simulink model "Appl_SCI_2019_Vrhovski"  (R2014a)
settings: Solver=ode45  StartTime=0.0  StopTime=1000  MaxStep=0.01  RelTol=1e-3
undefined symbols (not defined in the file): deg, H, kg, m, M, mm, N, rad, s, X, Y, Z
libraries: sm_lib x389, nesl_utility x69, simulink x7
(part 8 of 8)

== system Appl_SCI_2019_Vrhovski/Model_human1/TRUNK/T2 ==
  Mux : Mux  Inputs=3
  Pos X Converter : nesl_utility/PS-Simulink Converter  PhysicalDomain=network_engine_domain  SubClassName=ps_output  LeftPortType=input  RightPortType=output  PseudoPeriodic=off  Frequencies=[]  Unit=mm  AffineConversion=off
  Pos Y Converter : nesl_utility/PS-Simulink Converter  PhysicalDomain=network_engine_domain  SubClassName=ps_output  LeftPortType=input  RightPortType=output  PseudoPeriodic=off  Frequencies=[]  Unit=mm  AffineConversion=off
  Pos Z Converter2 : nesl_utility/PS-Simulink Converter  PhysicalDomain=network_engine_domain  SubClassName=ps_output  LeftPortType=input  RightPortType=output  PseudoPeriodic=off  Frequencies=[]  Unit=mm  AffineConversion=off
  Transform Sensor : sm_lib/Frames and Transforms/Transform Sensor  MeasurementFrame=World  SenseAngle=off  SenseAxis=off  SenseAngle1=off  SenseAngle2=off  SenseAngle3=off  SenseQ=off  SenseR=off  SenseOmegaX=off  SenseOmegaY=off  SenseOmegaZ=off  SenseOmega1=off  SenseOmega2=off  SenseOmega3=off  SenseQDot=off  SenseRDot=off  SenseAlphaX=off  SenseAlphaY=off  SenseAlphaZ=off  SenseAlpha1=off  SenseAlpha2=off  SenseAlpha3=off  SenseQDDot=off  SenseRDDot=off  SenseX=on  SenseY=on  SenseZ=on  SenseRad=on  SenseAzim=off  SenseDist=off  SenseInc=off  SenseXDot=off  SenseYDot=off  SenseZDot=off  SenseRadDot=off  SenseAzimDot=off  SenseDistDot=off  SenseIncDot=off  SenseXDDot=off  SenseYDDot=off  SenseZDDot=off  SenseRadDDot=off  SenseAzimDDot=off  SenseDistDDot=off  SenseIncDDot=off  BlockFunction=simmechanics.library.frames_transforms.transform_sensor
  base_coord_sys : PMIOPort  Port=1  Side=Left
  marker : PMIOPort  Port=2  Side=Left
  xyz : Outport
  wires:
  Mux/1 -> xyz/1
  Pos Y Converter/1 -> Mux/2
  Pos X Converter/1 -> Mux/1
  Pos Z Converter2/1 -> Mux/3
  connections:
  Transform Sensor/RConn3 -- Pos Y Converter/LConn1
  Pos X Converter/LConn1 -- Transform Sensor/RConn2
  Pos Z Converter2/LConn1 -- Transform Sensor/RConn4
  marker/RConn1 -- Transform Sensor/RConn1
  base_coord_sys/RConn1 -- Transform Sensor/LConn1

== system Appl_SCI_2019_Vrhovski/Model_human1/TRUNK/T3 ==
  Mux : Mux  Inputs=3
  Pos X Converter : nesl_utility/PS-Simulink Converter  PhysicalDomain=network_engine_domain  SubClassName=ps_output  LeftPortType=input  RightPortType=output  PseudoPeriodic=off  Frequencies=[]  Unit=mm  AffineConversion=off
  Pos Y Converter : nesl_utility/PS-Simulink Converter  PhysicalDomain=network_engine_domain  SubClassName=ps_output  LeftPortType=input  RightPortType=output  PseudoPeriodic=off  Frequencies=[]  Unit=mm  AffineConversion=off
  Pos Z Converter2 : nesl_utility/PS-Simulink Converter  PhysicalDomain=network_engine_domain  SubClassName=ps_output  LeftPortType=input  RightPortType=output  PseudoPeriodic=off  Frequencies=[]  Unit=mm  AffineConversion=off
  Transform Sensor : sm_lib/Frames and Transforms/Transform Sensor  MeasurementFrame=World  SenseAngle=off  SenseAxis=off  SenseAngle1=off  SenseAngle2=off  SenseAngle3=off  SenseQ=off  SenseR=off  SenseOmegaX=off  SenseOmegaY=off  SenseOmegaZ=off  SenseOmega1=off  SenseOmega2=off  SenseOmega3=off  SenseQDot=off  SenseRDot=off  SenseAlphaX=off  SenseAlphaY=off  SenseAlphaZ=off  SenseAlpha1=off  SenseAlpha2=off  SenseAlpha3=off  SenseQDDot=off  SenseRDDot=off  SenseX=on  SenseY=on  SenseZ=on  SenseRad=on  SenseAzim=off  SenseDist=off  SenseInc=off  SenseXDot=off  SenseYDot=off  SenseZDot=off  SenseRadDot=off  SenseAzimDot=off  SenseDistDot=off  SenseIncDot=off  SenseXDDot=off  SenseYDDot=off  SenseZDDot=off  SenseRadDDot=off  SenseAzimDDot=off  SenseDistDDot=off  SenseIncDDot=off  BlockFunction=simmechanics.library.frames_transforms.transform_sensor
  base_coord_sys : PMIOPort  Port=1  Side=Left
  marker : PMIOPort  Port=2  Side=Left
  xyz : Outport
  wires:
  Pos Z Converter2/1 -> Mux/3
  Pos X Converter/1 -> Mux/1
  Pos Y Converter/1 -> Mux/2
  Mux/1 -> xyz/1
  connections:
  base_coord_sys/RConn1 -- Transform Sensor/LConn1
  marker/RConn1 -- Transform Sensor/RConn1
  Pos Z Converter2/LConn1 -- Transform Sensor/RConn4
  Pos X Converter/LConn1 -- Transform Sensor/RConn2
  Transform Sensor/RConn3 -- Pos Y Converter/LConn1

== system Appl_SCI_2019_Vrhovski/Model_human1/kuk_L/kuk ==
  ReferenceFrame : sm_lib/Frames and Transforms/Reference Frame  BlockFunction=simmechanics.library.frames_transforms.reference_frame
  Solid : sm_lib/Body Elements/Solid  InertiaType=Custom  Mass=0  MassUnits=kg  CenterOfMass=[0 0 0]  CenterOfMassUnits=mm  MomentsOfInertia=[2897.1863857204326 1.8962829928219973 2897.1862300567827]  MomentsOfInertiaUnits=kg*mm^2  ProductsOfInertia=[0 0 -0.00027890183916846033]  ProductsOfInertiaUnits=kg*mm^2  DensityBased=on  Density=1000  DensityUnits=kg/(m^3)  GraphicType=FromGeometry  MarkerShape=Sphere  MarkerSize=10  MarkerSizeUnits=m  GraphicVisPropType=SimpleVisualProperties  GraphicDiffuseColor=[0.792156862745098 0.81960784313725488 0.93333333333333335]  GraphicSpecularColor=[0.5 0.5 0.5 1.0]  GraphicAmbientColor=[0.15 0.15 0.15 1.0]  GraphicEmissiveColor=[0.0 0.0 0.0 1.0]  GraphicShininess=75  GraphicOpacity=1  GeometryShape=Sphere  RectangleSize=[1 1]  RectangleSizeUnits=m  BrickDimensions=[1 1 1]  BrickDimensionUnits=m  CylinderRadius=1  CylinderRadiusUnits=m  CylinderLength=1  CylinderLengthUnits=m  SphereRadius=3  SphereRadiusUnits=cm  EllipsoidRadii=[1 1 1]  EllipsoidRadiiUnits=m  ExtrusionCrossSection=[1 1; -1 1; -1 -1; 1 -1]  ExtrusionCrossSectionUnits=m  ExtrusionLength=1  ExtrusionLengthUnits=m  PolygonNumSides=3  PolygonOuterRadius=1  PolygonOuterRadiusUnits=m  ExtGeomFileType=STL  ExtGeomFileName=Pod_Default_sldprt.STL  ExtGeomFileUnits=mm  RevolutionCrossSection=[1 1; 1 -1; 2 -1; 2 1]  RevolutionCrossSectionUnits=m  RevolutionExtent=Full  RevolutionAngle=180  RevolutionAngleUnits=deg  BlockFunction=simmechanics.library.body_elements.solid
  Transform : sm_lib/Frames and Transforms/Rigid Transform  TranslationMethod=None  TranslationLengthUnit=mm  TranslationStandardAxis=+Z  TranslationStandardOffset=100  TranslationCartesianOffset=[-2.2026824808563106e-13 549.99999999999943 3.4106051316484809e-13]  TranslationROffset=0  TranslationROffsetUnits=m  TranslationZOffset=0  TranslationZOffsetUnits=m  TranslationThetaOffset=0  TranslationThetaOffsetUnits=deg  RotationMethod=None  RotationAngleUnits=rad  RotationStandardAxis=+Z  RotationAngle=2.0943951023931962  RotationArbitraryAxis=[0.57735026918962595 -0.57735026918962618 0.57735026918962518]  FollAlignAxisA=+X  BaseAlignAxisA=+Y  FollAlignAxisB=+Y  BaseAlignAxisB=+Z  BlockFunction=simmechanics.library.frames_transforms.rigid_transform
  Transform1 : sm_lib/Frames and Transforms/Rigid Transform  TranslationMethod=StandardAxis  TranslationLengthUnit=mm  TranslationStandardAxis=+Z  TranslationStandardOffset=50  TranslationCartesianOffset=[1.3358203432289883e-12 0 -1.0913936421275139e-11]  TranslationROffset=0  TranslationROffsetUnits=m  TranslationZOffset=0  TranslationZOffsetUnits=m  TranslationThetaOffset=0  TranslationThetaOffsetUnits=deg  RotationMethod=None  RotationAngleUnits=rad  RotationStandardAxis=+X  RotationAngle=pi/2  RotationArbitraryAxis=[0 0 0]  FollAlignAxisA=+X  BaseAlignAxisA=+Y  FollAlignAxisB=+Y  BaseAlignAxisB=+Z  BlockFunction=simmechanics.library.frames_transforms.rigid_transform
  F : PMIOPort  Port=1  Side=Right
  B : PMIOPort  Port=2  Side=Left
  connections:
  Transform1/RConn1 -- F/RConn1
  Transform/RConn1 -- B/RConn1
  Solid/RConn1 -- ReferenceFrame/RConn1 -- Transform1/LConn1 -- Transform/LConn1

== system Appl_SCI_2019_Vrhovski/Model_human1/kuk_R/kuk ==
  ReferenceFrame : sm_lib/Frames and Transforms/Reference Frame  BlockFunction=simmechanics.library.frames_transforms.reference_frame
  Solid : sm_lib/Body Elements/Solid  InertiaType=Custom  Mass=0  MassUnits=kg  CenterOfMass=[0 0 0]  CenterOfMassUnits=mm  MomentsOfInertia=[2897.1863857204326 1.8962829928219973 2897.1862300567827]  MomentsOfInertiaUnits=kg*mm^2  ProductsOfInertia=[0 0 -0.00027890183916846033]  ProductsOfInertiaUnits=kg*mm^2  DensityBased=on  Density=1000  DensityUnits=kg/(m^3)  GraphicType=FromGeometry  MarkerShape=Sphere  MarkerSize=10  MarkerSizeUnits=m  GraphicVisPropType=SimpleVisualProperties  GraphicDiffuseColor=[0.792156862745098 0.81960784313725488 0.93333333333333335]  GraphicSpecularColor=[0.5 0.5 0.5 1.0]  GraphicAmbientColor=[0.15 0.15 0.15 1.0]  GraphicEmissiveColor=[0.0 0.0 0.0 1.0]  GraphicShininess=75  GraphicOpacity=1  GeometryShape=Sphere  RectangleSize=[1 1]  RectangleSizeUnits=m  BrickDimensions=[1 1 1]  BrickDimensionUnits=m  CylinderRadius=1  CylinderRadiusUnits=m  CylinderLength=1  CylinderLengthUnits=m  SphereRadius=3  SphereRadiusUnits=cm  EllipsoidRadii=[1 1 1]  EllipsoidRadiiUnits=m  ExtrusionCrossSection=[1 1; -1 1; -1 -1; 1 -1]  ExtrusionCrossSectionUnits=m  ExtrusionLength=1  ExtrusionLengthUnits=m  PolygonNumSides=3  PolygonOuterRadius=1  PolygonOuterRadiusUnits=m  ExtGeomFileType=STL  ExtGeomFileName=Pod_Default_sldprt.STL  ExtGeomFileUnits=mm  RevolutionCrossSection=[1 1; 1 -1; 2 -1; 2 1]  RevolutionCrossSectionUnits=m  RevolutionExtent=Full  RevolutionAngle=180  RevolutionAngleUnits=deg  BlockFunction=simmechanics.library.body_elements.solid
  Transform : sm_lib/Frames and Transforms/Rigid Transform  TranslationMethod=None  TranslationLengthUnit=mm  TranslationStandardAxis=+Z  TranslationStandardOffset=0  TranslationCartesianOffset=[-2.2026824808563106e-13 549.99999999999943 3.4106051316484809e-13]  TranslationROffset=0  TranslationROffsetUnits=m  TranslationZOffset=0  TranslationZOffsetUnits=m  TranslationThetaOffset=0  TranslationThetaOffsetUnits=deg  RotationMethod=None  RotationAngleUnits=rad  RotationStandardAxis=+Z  RotationAngle=2.0943951023931962  RotationArbitraryAxis=[0.57735026918962595 -0.57735026918962618 0.57735026918962518]  FollAlignAxisA=+X  BaseAlignAxisA=+Y  FollAlignAxisB=+Y  BaseAlignAxisB=+Z  BlockFunction=simmechanics.library.frames_transforms.rigid_transform
  Transform1 : sm_lib/Frames and Transforms/Rigid Transform  TranslationMethod=StandardAxis  TranslationLengthUnit=mm  TranslationStandardAxis=+Z  TranslationStandardOffset=50  TranslationCartesianOffset=[1.3358203432289883e-12 0 -1.0913936421275139e-11]  TranslationROffset=0  TranslationROffsetUnits=m  TranslationZOffset=0  TranslationZOffsetUnits=m  TranslationThetaOffset=0  TranslationThetaOffsetUnits=deg  RotationMethod=None  RotationAngleUnits=rad  RotationStandardAxis=+X  RotationAngle=pi/2  RotationArbitraryAxis=[0 0 0]  FollAlignAxisA=+X  BaseAlignAxisA=+Y  FollAlignAxisB=+Y  BaseAlignAxisB=+Z  BlockFunction=simmechanics.library.frames_transforms.rigid_transform
  F : PMIOPort  Port=1  Side=Right
  B : PMIOPort  Port=2  Side=Left
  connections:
  Transform/LConn1 -- Transform1/LConn1 -- ReferenceFrame/RConn1 -- Solid/RConn1
  Transform/RConn1 -- B/RConn1
  Transform1/RConn1 -- F/RConn1

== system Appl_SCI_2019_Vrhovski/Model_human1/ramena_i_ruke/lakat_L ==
  ReferenceFrame : sm_lib/Frames and Transforms/Reference Frame  BlockFunction=simmechanics.library.frames_transforms.reference_frame
  Solid : sm_lib/Body Elements/Solid  InertiaType=Custom  Mass=0  MassUnits=kg  CenterOfMass=[0 0 0]  CenterOfMassUnits=mm  MomentsOfInertia=[2897.1863857204326 1.8962829928219973 2897.1862300567827]  MomentsOfInertiaUnits=kg*mm^2  ProductsOfInertia=[0 0 -0.00027890183916846033]  ProductsOfInertiaUnits=kg*mm^2  DensityBased=on  Density=1000  DensityUnits=kg/(m^3)  GraphicType=FromGeometry  MarkerShape=Sphere  MarkerSize=10  MarkerSizeUnits=m  GraphicVisPropType=SimpleVisualProperties  GraphicDiffuseColor=[0.792156862745098 0.81960784313725488 0.93333333333333335]  GraphicSpecularColor=[0.5 0.5 0.5 1.0]  GraphicAmbientColor=[0.15 0.15 0.15 1.0]  GraphicEmissiveColor=[0.0 0.0 0.0 1.0]  GraphicShininess=75  GraphicOpacity=1  GeometryShape=Sphere  RectangleSize=[1 1]  RectangleSizeUnits=m  BrickDimensions=[1 1 1]  BrickDimensionUnits=m  CylinderRadius=1  CylinderRadiusUnits=m  CylinderLength=1  CylinderLengthUnits=m  SphereRadius=3  SphereRadiusUnits=cm  EllipsoidRadii=[1 1 1]  EllipsoidRadiiUnits=m  ExtrusionCrossSection=[1 1; -1 1; -1 -1; 1 -1]  ExtrusionCrossSectionUnits=m  ExtrusionLength=1  ExtrusionLengthUnits=m  PolygonNumSides=3  PolygonOuterRadius=1  PolygonOuterRadiusUnits=m  ExtGeomFileType=STL  ExtGeomFileName=Pod_Default_sldprt.STL  ExtGeomFileUnits=mm  RevolutionCrossSection=[1 1; 1 -1; 2 -1; 2 1]  RevolutionCrossSectionUnits=m  RevolutionExtent=Full  RevolutionAngle=180  RevolutionAngleUnits=deg  BlockFunction=simmechanics.library.body_elements.solid
  Transform : sm_lib/Frames and Transforms/Rigid Transform  TranslationMethod=None  TranslationLengthUnit=mm  TranslationStandardAxis=+Z  TranslationStandardOffset=0  TranslationCartesianOffset=[-2.2026824808563106e-13 549.99999999999943 3.4106051316484809e-13]  TranslationROffset=0  TranslationROffsetUnits=m  TranslationZOffset=0  TranslationZOffsetUnits=m  TranslationThetaOffset=0  TranslationThetaOffsetUnits=deg  RotationMethod=None  RotationAngleUnits=rad  RotationStandardAxis=+Z  RotationAngle=2.0943951023931962  RotationArbitraryAxis=[0.57735026918962595 -0.57735026918962618 0.57735026918962518]  FollAlignAxisA=+X  BaseAlignAxisA=+Y  FollAlignAxisB=+Y  BaseAlignAxisB=+Z  BlockFunction=simmechanics.library.frames_transforms.rigid_transform
  Transform1 : sm_lib/Frames and Transforms/Rigid Transform  TranslationMethod=None  TranslationLengthUnit=mm  TranslationStandardAxis=+Z  TranslationStandardOffset=0  TranslationCartesianOffset=[1.3358203432289883e-12 0 -1.0913936421275139e-11]  TranslationROffset=0  TranslationROffsetUnits=m  TranslationZOffset=0  TranslationZOffsetUnits=m  TranslationThetaOffset=0  TranslationThetaOffsetUnits=deg  RotationMethod=None  RotationAngleUnits=rad  RotationStandardAxis=+X  RotationAngle=pi/2  RotationArbitraryAxis=[0 0 0]  FollAlignAxisA=+X  BaseAlignAxisA=+Y  FollAlignAxisB=+Y  BaseAlignAxisB=+Z  BlockFunction=simmechanics.library.frames_transforms.rigid_transform
  F : PMIOPort  Port=1  Side=Right
  B : PMIOPort  Port=2  Side=Left
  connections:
  Transform/LConn1 -- Transform1/LConn1 -- ReferenceFrame/RConn1 -- Solid/RConn1
  Transform/RConn1 -- B/RConn1
  Transform1/RConn1 -- F/RConn1

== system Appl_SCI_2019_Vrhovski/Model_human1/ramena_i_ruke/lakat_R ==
  ReferenceFrame : sm_lib/Frames and Transforms/Reference Frame  BlockFunction=simmechanics.library.frames_transforms.reference_frame
  Solid : sm_lib/Body Elements/Solid  InertiaType=Custom  Mass=0  MassUnits=kg  CenterOfMass=[0 0 0]  CenterOfMassUnits=mm  MomentsOfInertia=[2897.1863857204326 1.8962829928219973 2897.1862300567827]  MomentsOfInertiaUnits=kg*mm^2  ProductsOfInertia=[0 0 -0.00027890183916846033]  ProductsOfInertiaUnits=kg*mm^2  DensityBased=on  Density=1000  DensityUnits=kg/(m^3)  GraphicType=FromGeometry  MarkerShape=Sphere  MarkerSize=10  MarkerSizeUnits=m  GraphicVisPropType=SimpleVisualProperties  GraphicDiffuseColor=[0.792156862745098 0.81960784313725488 0.93333333333333335]  GraphicSpecularColor=[0.5 0.5 0.5 1.0]  GraphicAmbientColor=[0.15 0.15 0.15 1.0]  GraphicEmissiveColor=[0.0 0.0 0.0 1.0]  GraphicShininess=75  GraphicOpacity=1  GeometryShape=Sphere  RectangleSize=[1 1]  RectangleSizeUnits=m  BrickDimensions=[1 1 1]  BrickDimensionUnits=m  CylinderRadius=1  CylinderRadiusUnits=m  CylinderLength=1  CylinderLengthUnits=m  SphereRadius=3  SphereRadiusUnits=cm  EllipsoidRadii=[1 1 1]  EllipsoidRadiiUnits=m  ExtrusionCrossSection=[1 1; -1 1; -1 -1; 1 -1]  ExtrusionCrossSectionUnits=m  ExtrusionLength=1  ExtrusionLengthUnits=m  PolygonNumSides=3  PolygonOuterRadius=1  PolygonOuterRadiusUnits=m  ExtGeomFileType=STL  ExtGeomFileName=Pod_Default_sldprt.STL  ExtGeomFileUnits=mm  RevolutionCrossSection=[1 1; 1 -1; 2 -1; 2 1]  RevolutionCrossSectionUnits=m  RevolutionExtent=Full  RevolutionAngle=180  RevolutionAngleUnits=deg  BlockFunction=simmechanics.library.body_elements.solid
  Transform : sm_lib/Frames and Transforms/Rigid Transform  TranslationMethod=None  TranslationLengthUnit=mm  TranslationStandardAxis=+Z  TranslationStandardOffset=0  TranslationCartesianOffset=[-2.2026824808563106e-13 549.99999999999943 3.4106051316484809e-13]  TranslationROffset=0  TranslationROffsetUnits=m  TranslationZOffset=0  TranslationZOffsetUnits=m  TranslationThetaOffset=0  TranslationThetaOffsetUnits=deg  RotationMethod=None  RotationAngleUnits=rad  RotationStandardAxis=+Z  RotationAngle=2.0943951023931962  RotationArbitraryAxis=[0.57735026918962595 -0.57735026918962618 0.57735026918962518]  FollAlignAxisA=+X  BaseAlignAxisA=+Y  FollAlignAxisB=+Y  BaseAlignAxisB=+Z  BlockFunction=simmechanics.library.frames_transforms.rigid_transform
  Transform1 : sm_lib/Frames and Transforms/Rigid Transform  TranslationMethod=None  TranslationLengthUnit=mm  TranslationStandardAxis=+Z  TranslationStandardOffset=0  TranslationCartesianOffset=[1.3358203432289883e-12 0 -1.0913936421275139e-11]  TranslationROffset=0  TranslationROffsetUnits=m  TranslationZOffset=0  TranslationZOffsetUnits=m  TranslationThetaOffset=0  TranslationThetaOffsetUnits=deg  RotationMethod=None  RotationAngleUnits=rad  RotationStandardAxis=+X  RotationAngle=pi/2  RotationArbitraryAxis=[0 0 0]  FollAlignAxisA=+X  BaseAlignAxisA=+Y  FollAlignAxisB=+Y  BaseAlignAxisB=+Z  BlockFunction=simmechanics.library.frames_transforms.rigid_transform
  F : PMIOPort  Port=1  Side=Right
  B : PMIOPort  Port=2  Side=Left
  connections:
  Transform1/RConn1 -- F/RConn1
  Transform/RConn1 -- B/RConn1
  Solid/RConn1 -- ReferenceFrame/RConn1 -- Transform1/LConn1 -- Transform/LConn1

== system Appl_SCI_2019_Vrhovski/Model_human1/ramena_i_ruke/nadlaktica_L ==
  ReferenceFrame : sm_lib/Frames and Transforms/Reference Frame  BlockFunction=simmechanics.library.frames_transforms.reference_frame
  Solid : sm_lib/Body Elements/Solid  InertiaType=Custom  Mass=0.03*M  MassUnits=kg  CenterOfMass=[0 0 0]  CenterOfMassUnits=mm  MomentsOfInertia=[2897.1863857204326 1.8962829928219973 2897.1862300567827]  MomentsOfInertiaUnits=kg*mm^2  ProductsOfInertia=[0 0 -0.00027890183916846033]  ProductsOfInertiaUnits=kg*mm^2  DensityBased=on  Density=1000  DensityUnits=kg/(m^3)  GraphicType=FromGeometry  MarkerShape=Sphere  MarkerSize=10  MarkerSizeUnits=m  GraphicVisPropType=SimpleVisualProperties  GraphicDiffuseColor=[0.792156862745098 0.81960784313725488 0.93333333333333335]  GraphicSpecularColor=[0.5 0.5 0.5 1.0]  GraphicAmbientColor=[0.15 0.15 0.15 1.0]  GraphicEmissiveColor=[0.0 0.0 0.0 1.0]  GraphicShininess=75  GraphicOpacity=1  GeometryShape=Ellipsoid  RectangleSize=[1 1]  RectangleSizeUnits=m  BrickDimensions=[1 1 1]  BrickDimensionUnits=m  CylinderRadius=2.5  CylinderRadiusUnits=cm  CylinderLength=25  CylinderLengthUnits=cm  SphereRadius=5  SphereRadiusUnits=cm  EllipsoidRadii=[40 40 125]  EllipsoidRadiiUnits=mm  ExtrusionCrossSection=[1 1; -1 1; -1 -1; 1 -1]  ExtrusionCrossSectionUnits=m  ExtrusionLength=1  ExtrusionLengthUnits=m  PolygonNumSides=3  PolygonOuterRadius=1  PolygonOuterRadiusUnits=m  ExtGeomFileType=STL  ExtGeomFileName=Pod_Default_sldprt.STL  ExtGeomFileUnits=mm  RevolutionCrossSection=[1 1; 1 -1; 2 -1; 2 1]  RevolutionCrossSectionUnits=m  RevolutionExtent=Full  RevolutionAngle=180  RevolutionAngleUnits=deg  BlockFunction=simmechanics.library.body_elements.solid
  Transform1 : sm_lib/Frames and Transforms/Rigid Transform  TranslationMethod=StandardAxis  TranslationLengthUnit=mm  TranslationStandardAxis=+Z  TranslationStandardOffset=125  TranslationCartesianOffset=[1.3358203432289883e-12 650.00000000000045 -1.0913936421275139e-11]  TranslationROffset=0  TranslationROffsetUnits=m  TranslationZOffset=0  TranslationZOffsetUnits=m  TranslationThetaOffset=0  TranslationThetaOffsetUnits=deg  RotationMethod=None  RotationAngleUnits=rad  RotationStandardAxis=+Z  RotationAngle=0  RotationArbitraryAxis=[0 0 0]  FollAlignAxisA=+X  BaseAlignAxisA=+Y  FollAlignAxisB=+Y  BaseAlignAxisB=+Z  BlockFunction=simmechanics.library.frames_transforms.rigid_transform
  Transform2 : sm_lib/Frames and Transforms/Rigid Transform  TranslationMethod=StandardAxis  TranslationLengthUnit=mm  TranslationStandardAxis=-Z  TranslationStandardOffset=125  TranslationCartesianOffset=[-2.2026824808563106e-13 549.99999999999943 3.4106051316484809e-13]  TranslationROffset=0  TranslationROffsetUnits=m  TranslationZOffset=0  TranslationZOffsetUnits=m  TranslationThetaOffset=0  TranslationThetaOffsetUnits=deg  RotationMethod=None  RotationAngleUnits=rad  RotationStandardAxis=+X  RotationAngle=pi/2  RotationArbitraryAxis=[0.57735026918962595 -0.57735026918962618 0.57735026918962518]  FollAlignAxisA=+X  BaseAlignAxisA=+Y  FollAlignAxisB=+Y  BaseAlignAxisB=+Z  BlockFunction=simmechanics.library.frames_transforms.rigid_transform
  F : PMIOPort  Port=1  Side=Right
  B : PMIOPort  Port=2  Side=Left
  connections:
  Transform2/LConn1 -- Transform1/LConn1 -- Solid/RConn1 -- ReferenceFrame/RConn1
  Transform1/RConn1 -- F/RConn1
  B/RConn1 -- Transform2/RConn1

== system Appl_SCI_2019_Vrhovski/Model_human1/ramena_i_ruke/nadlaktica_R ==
  ReferenceFrame : sm_lib/Frames and Transforms/Reference Frame  BlockFunction=simmechanics.library.frames_transforms.reference_frame
  Solid : sm_lib/Body Elements/Solid  InertiaType=Custom  Mass=0.03*M  MassUnits=kg  CenterOfMass=[0 0 0]  CenterOfMassUnits=mm  MomentsOfInertia=[2897.1863857204326 1.8962829928219973 2897.1862300567827]  MomentsOfInertiaUnits=kg*mm^2  ProductsOfInertia=[0 0 -0.00027890183916846033]  ProductsOfInertiaUnits=kg*mm^2  DensityBased=on  Density=1000  DensityUnits=kg/(m^3)  GraphicType=FromGeometry  MarkerShape=Sphere  MarkerSize=10  MarkerSizeUnits=m  GraphicVisPropType=SimpleVisualProperties  GraphicDiffuseColor=[0.792156862745098 0.81960784313725488 0.93333333333333335]  GraphicSpecularColor=[0.5 0.5 0.5 1.0]  GraphicAmbientColor=[0.15 0.15 0.15 1.0]  GraphicEmissiveColor=[0.0 0.0 0.0 1.0]  GraphicShininess=75  GraphicOpacity=1  GeometryShape=Ellipsoid  RectangleSize=[1 1]  RectangleSizeUnits=m  BrickDimensions=[1 1 1]  BrickDimensionUnits=m  CylinderRadius=2.5  CylinderRadiusUnits=cm  CylinderLength=25  CylinderLengthUnits=cm  SphereRadius=5  SphereRadiusUnits=cm  EllipsoidRadii=[40 40 125]  EllipsoidRadiiUnits=mm  ExtrusionCrossSection=[1 1; -1 1; -1 -1; 1 -1]  ExtrusionCrossSectionUnits=m  ExtrusionLength=1  ExtrusionLengthUnits=m  PolygonNumSides=3  PolygonOuterRadius=1  PolygonOuterRadiusUnits=m  ExtGeomFileType=STL  ExtGeomFileName=Pod_Default_sldprt.STL  ExtGeomFileUnits=mm  RevolutionCrossSection=[1 1; 1 -1; 2 -1; 2 1]  RevolutionCrossSectionUnits=m  RevolutionExtent=Full  RevolutionAngle=180  RevolutionAngleUnits=deg  BlockFunction=simmechanics.library.body_elements.solid
  Transform1 : sm_lib/Frames and Transforms/Rigid Transform  TranslationMethod=StandardAxis  TranslationLengthUnit=mm  TranslationStandardAxis=+Z  TranslationStandardOffset=125  TranslationCartesianOffset=[1.3358203432289883e-12 650.00000000000045 -1.0913936421275139e-11]  TranslationROffset=0  TranslationROffsetUnits=m  TranslationZOffset=0  TranslationZOffsetUnits=m  TranslationThetaOffset=0  TranslationThetaOffsetUnits=deg  RotationMethod=None  RotationAngleUnits=rad  RotationStandardAxis=+Z  RotationAngle=0  RotationArbitraryAxis=[0 0 0]  FollAlignAxisA=+X  BaseAlignAxisA=+Y  FollAlignAxisB=+Y  BaseAlignAxisB=+Z  BlockFunction=simmechanics.library.frames_transforms.rigid_transform
  Transform2 : sm_lib/Frames and Transforms/Rigid Transform  TranslationMethod=StandardAxis  TranslationLengthUnit=mm  TranslationStandardAxis=-Z  TranslationStandardOffset=125  TranslationCartesianOffset=[-2.2026824808563106e-13 549.99999999999943 3.4106051316484809e-13]  TranslationROffset=0  TranslationROffsetUnits=m  TranslationZOffset=0  TranslationZOffsetUnits=m  TranslationThetaOffset=0  TranslationThetaOffsetUnits=deg  RotationMethod=None  RotationAngleUnits=rad  RotationStandardAxis=+X  RotationAngle=pi/2  RotationArbitraryAxis=[0.57735026918962595 -0.57735026918962618 0.57735026918962518]  FollAlignAxisA=+X  BaseAlignAxisA=+Y  FollAlignAxisB=+Y  BaseAlignAxisB=+Z  BlockFunction=simmechanics.library.frames_transforms.rigid_transform
  F : PMIOPort  Port=1  Side=Right
  B : PMIOPort  Port=2  Side=Left
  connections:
  B/RConn1 -- Transform2/RConn1
  Transform1/RConn1 -- F/RConn1
  ReferenceFrame/RConn1 -- Solid/RConn1 -- Transform1/LConn1 -- Transform2/LConn1

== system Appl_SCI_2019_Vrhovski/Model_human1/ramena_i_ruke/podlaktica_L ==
  ReferenceFrame : sm_lib/Frames and Transforms/Reference Frame  BlockFunction=simmechanics.library.frames_transforms.reference_frame
  Solid : sm_lib/Body Elements/Solid  InertiaType=Custom  Mass=0.0194*M  MassUnits=kg  CenterOfMass=[0 0 0]  CenterOfMassUnits=mm  MomentsOfInertia=[2897.1863857204326 1.8962829928219973 2897.1862300567827]  MomentsOfInertiaUnits=kg*mm^2  ProductsOfInertia=[0 0 -0.00027890183916846033]  ProductsOfInertiaUnits=kg*mm^2  DensityBased=on  Density=1000  DensityUnits=kg/(m^3)  GraphicType=FromGeometry  MarkerShape=Sphere  MarkerSize=10  MarkerSizeUnits=m  GraphicVisPropType=SimpleVisualProperties  GraphicDiffuseColor=[0.792156862745098 0.81960784313725488 0.93333333333333335]  GraphicSpecularColor=[0.5 0.5 0.5 1.0]  GraphicAmbientColor=[0.15 0.15 0.15 1.0]  GraphicEmissiveColor=[0.0 0.0 0.0 1.0]  GraphicShininess=75  GraphicOpacity=1  GeometryShape=Ellipsoid  RectangleSize=[1 1]  RectangleSizeUnits=m  BrickDimensions=[1 1 1]  BrickDimensionUnits=m  CylinderRadius=2.5  CylinderRadiusUnits=cm  CylinderLength=20  CylinderLengthUnits=cm  SphereRadius=5  SphereRadiusUnits=cm  EllipsoidRadii=[30 30 100]  EllipsoidRadiiUnits=mm  ExtrusionCrossSection=[1 1; -1 1; -1 -1; 1 -1]  ExtrusionCrossSectionUnits=m  ExtrusionLength=1  ExtrusionLengthUnits=m  PolygonNumSides=3  PolygonOuterRadius=1  PolygonOuterRadiusUnits=m  ExtGeomFileType=STL  ExtGeomFileName=Pod_Default_sldprt.STL  ExtGeomFileUnits=mm  RevolutionCrossSection=[1 1; 1 -1; 2 -1; 2 1]  RevolutionCrossSectionUnits=m  RevolutionExtent=Full  RevolutionAngle=180  RevolutionAngleUnits=deg  BlockFunction=simmechanics.library.body_elements.solid
  Transform1 : sm_lib/Frames and Transforms/Rigid Transform  TranslationMethod=StandardAxis  TranslationLengthUnit=mm  TranslationStandardAxis=+Z  TranslationStandardOffset=100  TranslationCartesianOffset=[1.3358203432289883e-12 650.00000000000045 -1.0913936421275139e-11]  TranslationROffset=0  TranslationROffsetUnits=m  TranslationZOffset=0  TranslationZOffsetUnits=m  TranslationThetaOffset=0  TranslationThetaOffsetUnits=deg  RotationMethod=None  RotationAngleUnits=rad  RotationStandardAxis=+Z  RotationAngle=0  RotationArbitraryAxis=[0 0 0]  FollAlignAxisA=+X  BaseAlignAxisA=+Y  FollAlignAxisB=+Y  BaseAlignAxisB=+Z  BlockFunction=simmechanics.library.frames_transforms.rigid_transform
  Transform2 : sm_lib/Frames and Transforms/Rigid Transform  TranslationMethod=StandardAxis  TranslationLengthUnit=mm  TranslationStandardAxis=-Z  TranslationStandardOffset=100  TranslationCartesianOffset=[-2.2026824808563106e-13 549.99999999999943 3.4106051316484809e-13]  TranslationROffset=0  TranslationROffsetUnits=m  TranslationZOffset=0  TranslationZOffsetUnits=m  TranslationThetaOffset=0  TranslationThetaOffsetUnits=deg  RotationMethod=None  RotationAngleUnits=rad  RotationStandardAxis=+X  RotationAngle=pi/2  RotationArbitraryAxis=[0.57735026918962595 -0.57735026918962618 0.57735026918962518]  FollAlignAxisA=+X  BaseAlignAxisA=+Y  FollAlignAxisB=+Y  BaseAlignAxisB=+Z  BlockFunction=simmechanics.library.frames_transforms.rigid_transform
  F : PMIOPort  Port=1  Side=Right
  B : PMIOPort  Port=2  Side=Left
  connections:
  B/RConn1 -- Transform2/RConn1
  Transform1/RConn1 -- F/RConn1
  ReferenceFrame/RConn1 -- Solid/RConn1 -- Transform1/LConn1 -- Transform2/LConn1

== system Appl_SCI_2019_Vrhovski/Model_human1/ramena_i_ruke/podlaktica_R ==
  ReferenceFrame : sm_lib/Frames and Transforms/Reference Frame  BlockFunction=simmechanics.library.frames_transforms.reference_frame
  Solid : sm_lib/Body Elements/Solid  InertiaType=Custom  Mass=0.0194*M  MassUnits=kg  CenterOfMass=[0 0 0]  CenterOfMassUnits=mm  MomentsOfInertia=[2897.1863857204326 1.8962829928219973 2897.1862300567827]  MomentsOfInertiaUnits=kg*mm^2  ProductsOfInertia=[0 0 -0.00027890183916846033]  ProductsOfInertiaUnits=kg*mm^2  DensityBased=on  Density=1000  DensityUnits=kg/(m^3)  GraphicType=FromGeometry  MarkerShape=Sphere  MarkerSize=10  MarkerSizeUnits=m  GraphicVisPropType=SimpleVisualProperties  GraphicDiffuseColor=[0.792156862745098 0.81960784313725488 0.93333333333333335]  GraphicSpecularColor=[0.5 0.5 0.5 1.0]  GraphicAmbientColor=[0.15 0.15 0.15 1.0]  GraphicEmissiveColor=[0.0 0.0 0.0 1.0]  GraphicShininess=75  GraphicOpacity=1  GeometryShape=Ellipsoid  RectangleSize=[1 1]  RectangleSizeUnits=m  BrickDimensions=[1 1 1]  BrickDimensionUnits=m  CylinderRadius=2.5  CylinderRadiusUnits=cm  CylinderLength=20  CylinderLengthUnits=cm  SphereRadius=5  SphereRadiusUnits=cm  EllipsoidRadii=[30 30 100]  EllipsoidRadiiUnits=mm  ExtrusionCrossSection=[1 1; -1 1; -1 -1; 1 -1]  ExtrusionCrossSectionUnits=m  ExtrusionLength=1  ExtrusionLengthUnits=m  PolygonNumSides=3  PolygonOuterRadius=1  PolygonOuterRadiusUnits=m  ExtGeomFileType=STL  ExtGeomFileName=Pod_Default_sldprt.STL  ExtGeomFileUnits=mm  RevolutionCrossSection=[1 1; 1 -1; 2 -1; 2 1]  RevolutionCrossSectionUnits=m  RevolutionExtent=Full  RevolutionAngle=180  RevolutionAngleUnits=deg  BlockFunction=simmechanics.library.body_elements.solid
  Transform1 : sm_lib/Frames and Transforms/Rigid Transform  TranslationMethod=StandardAxis  TranslationLengthUnit=mm  TranslationStandardAxis=+Z  TranslationStandardOffset=100  TranslationCartesianOffset=[1.3358203432289883e-12 650.00000000000045 -1.0913936421275139e-11]  TranslationROffset=0  TranslationROffsetUnits=m  TranslationZOffset=0  TranslationZOffsetUnits=m  TranslationThetaOffset=0  TranslationThetaOffsetUnits=deg  RotationMethod=None  RotationAngleUnits=rad  RotationStandardAxis=+Z  RotationAngle=0  RotationArbitraryAxis=[0 0 0]  FollAlignAxisA=+X  BaseAlignAxisA=+Y  FollAlignAxisB=+Y  BaseAlignAxisB=+Z  BlockFunction=simmechanics.library.frames_transforms.rigid_transform
  Transform2 : sm_lib/Frames and Transforms/Rigid Transform  TranslationMethod=StandardAxis  TranslationLengthUnit=mm  TranslationStandardAxis=-Z  TranslationStandardOffset=100  TranslationCartesianOffset=[-2.2026824808563106e-13 549.99999999999943 3.4106051316484809e-13]  TranslationROffset=0  TranslationROffsetUnits=m  TranslationZOffset=0  TranslationZOffsetUnits=m  TranslationThetaOffset=0  TranslationThetaOffsetUnits=deg  RotationMethod=None  RotationAngleUnits=rad  RotationStandardAxis=+X  RotationAngle=pi/2  RotationArbitraryAxis=[0.57735026918962595 -0.57735026918962618 0.57735026918962518]  FollAlignAxisA=+X  BaseAlignAxisA=+Y  FollAlignAxisB=+Y  BaseAlignAxisB=+Z  BlockFunction=simmechanics.library.frames_transforms.rigid_transform
  F : PMIOPort  Port=1  Side=Right
  B : PMIOPort  Port=2  Side=Left
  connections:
  Transform2/LConn1 -- Transform1/LConn1 -- Solid/RConn1 -- ReferenceFrame/RConn1
  Transform1/RConn1 -- F/RConn1
  B/RConn1 -- Transform2/RConn1

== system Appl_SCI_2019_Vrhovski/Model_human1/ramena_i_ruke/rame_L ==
  ReferenceFrame : sm_lib/Frames and Transforms/Reference Frame  BlockFunction=simmechanics.library.frames_transforms.reference_frame
  Solid : sm_lib/Body Elements/Solid  InertiaType=Custom  Mass=0  MassUnits=kg  CenterOfMass=[0 0 0]  CenterOfMassUnits=mm  MomentsOfInertia=[2897.1863857204326 1.8962829928219973 2897.1862300567827]  MomentsOfInertiaUnits=kg*mm^2  ProductsOfInertia=[0 0 -0.00027890183916846033]  ProductsOfInertiaUnits=kg*mm^2  DensityBased=on  Density=1000  DensityUnits=kg/(m^3)  GraphicType=FromGeometry  MarkerShape=Sphere  MarkerSize=10  MarkerSizeUnits=m  GraphicVisPropType=SimpleVisualProperties  GraphicDiffuseColor=[0.792156862745098 0.81960784313725488 0.93333333333333335]  GraphicSpecularColor=[0.5 0.5 0.5 1.0]  GraphicAmbientColor=[0.15 0.15 0.15 1.0]  GraphicEmissiveColor=[0.0 0.0 0.0 1.0]  GraphicShininess=75  GraphicOpacity=1  GeometryShape=Sphere  RectangleSize=[1 1]  RectangleSizeUnits=m  BrickDimensions=[1 1 1]  BrickDimensionUnits=m  CylinderRadius=1  CylinderRadiusUnits=m  CylinderLength=1  CylinderLengthUnits=m  SphereRadius=3  SphereRadiusUnits=cm  EllipsoidRadii=[1 1 1]  EllipsoidRadiiUnits=m  ExtrusionCrossSection=[1 1; -1 1; -1 -1; 1 -1]  ExtrusionCrossSectionUnits=m  ExtrusionLength=1  ExtrusionLengthUnits=m  PolygonNumSides=3  PolygonOuterRadius=1  PolygonOuterRadiusUnits=m  ExtGeomFileType=STL  ExtGeomFileName=Pod_Default_sldprt.STL  ExtGeomFileUnits=mm  RevolutionCrossSection=[1 1; 1 -1; 2 -1; 2 1]  RevolutionCrossSectionUnits=m  RevolutionExtent=Full  RevolutionAngle=180  RevolutionAngleUnits=deg  BlockFunction=simmechanics.library.body_elements.solid
  Transform : sm_lib/Frames and Transforms/Rigid Transform  TranslationMethod=None  TranslationLengthUnit=mm  TranslationStandardAxis=+Z  TranslationStandardOffset=0  TranslationCartesianOffset=[-2.2026824808563106e-13 549.99999999999943 3.4106051316484809e-13]  TranslationROffset=0  TranslationROffsetUnits=m  TranslationZOffset=0  TranslationZOffsetUnits=m  TranslationThetaOffset=0  TranslationThetaOffsetUnits=deg  RotationMethod=None  RotationAngleUnits=rad  RotationStandardAxis=+Z  RotationAngle=2.0943951023931962  RotationArbitraryAxis=[0.57735026918962595 -0.57735026918962618 0.57735026918962518]  FollAlignAxisA=+X  BaseAlignAxisA=+Y  FollAlignAxisB=+Y  BaseAlignAxisB=+Z  BlockFunction=simmechanics.library.frames_transforms.rigid_transform
  Transform1 : sm_lib/Frames and Transforms/Rigid Transform  TranslationMethod=None  TranslationLengthUnit=mm  TranslationStandardAxis=+Z  TranslationStandardOffset=0  TranslationCartesianOffset=[1.3358203432289883e-12 0 -1.0913936421275139e-11]  TranslationROffset=0  TranslationROffsetUnits=m  TranslationZOffset=0  TranslationZOffsetUnits=m  TranslationThetaOffset=0  TranslationThetaOffsetUnits=deg  RotationMethod=None  RotationAngleUnits=rad  RotationStandardAxis=+X  RotationAngle=pi/2  RotationArbitraryAxis=[0 0 0]  FollAlignAxisA=+X  BaseAlignAxisA=+Y  FollAlignAxisB=+Y  BaseAlignAxisB=+Z  BlockFunction=simmechanics.library.frames_transforms.rigid_transform
  F : PMIOPort  Port=1  Side=Right
  B : PMIOPort  Port=2  Side=Left
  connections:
  Transform1/RConn1 -- F/RConn1
  Transform/RConn1 -- B/RConn1
  Solid/RConn1 -- ReferenceFrame/RConn1 -- Transform1/LConn1 -- Transform/LConn1

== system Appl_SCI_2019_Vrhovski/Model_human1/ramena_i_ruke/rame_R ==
  ReferenceFrame : sm_lib/Frames and Transforms/Reference Frame  BlockFunction=simmechanics.library.frames_transforms.reference_frame
  Solid : sm_lib/Body Elements/Solid  InertiaType=Custom  Mass=0  MassUnits=kg  CenterOfMass=[0 0 0]  CenterOfMassUnits=mm  MomentsOfInertia=[2897.1863857204326 1.8962829928219973 2897.1862300567827]  MomentsOfInertiaUnits=kg*mm^2  ProductsOfInertia=[0 0 -0.00027890183916846033]  ProductsOfInertiaUnits=kg*mm^2  DensityBased=on  Density=1000  DensityUnits=kg/(m^3)  GraphicType=FromGeometry  MarkerShape=Sphere  MarkerSize=10  MarkerSizeUnits=m  GraphicVisPropType=SimpleVisualProperties  GraphicDiffuseColor=[0.792156862745098 0.81960784313725488 0.93333333333333335]  GraphicSpecularColor=[0.5 0.5 0.5 1.0]  GraphicAmbientColor=[0.15 0.15 0.15 1.0]  GraphicEmissiveColor=[0.0 0.0 0.0 1.0]  GraphicShininess=75  GraphicOpacity=1  GeometryShape=Sphere  RectangleSize=[1 1]  RectangleSizeUnits=m  BrickDimensions=[1 1 1]  BrickDimensionUnits=m  CylinderRadius=1  CylinderRadiusUnits=m  CylinderLength=1  CylinderLengthUnits=m  SphereRadius=3  SphereRadiusUnits=cm  EllipsoidRadii=[1 1 1]  EllipsoidRadiiUnits=m  ExtrusionCrossSection=[1 1; -1 1; -1 -1; 1 -1]  ExtrusionCrossSectionUnits=m  ExtrusionLength=1  ExtrusionLengthUnits=m  PolygonNumSides=3  PolygonOuterRadius=1  PolygonOuterRadiusUnits=m  ExtGeomFileType=STL  ExtGeomFileName=Pod_Default_sldprt.STL  ExtGeomFileUnits=mm  RevolutionCrossSection=[1 1; 1 -1; 2 -1; 2 1]  RevolutionCrossSectionUnits=m  RevolutionExtent=Full  RevolutionAngle=180  RevolutionAngleUnits=deg  BlockFunction=simmechanics.library.body_elements.solid
  Transform : sm_lib/Frames and Transforms/Rigid Transform  TranslationMethod=None  TranslationLengthUnit=mm  TranslationStandardAxis=+Z  TranslationStandardOffset=0  TranslationCartesianOffset=[-2.2026824808563106e-13 549.99999999999943 3.4106051316484809e-13]  TranslationROffset=0  TranslationROffsetUnits=m  TranslationZOffset=0  TranslationZOffsetUnits=m  TranslationThetaOffset=0  TranslationThetaOffsetUnits=deg  RotationMethod=None  RotationAngleUnits=rad  RotationStandardAxis=+Z  RotationAngle=2.0943951023931962  RotationArbitraryAxis=[0.57735026918962595 -0.57735026918962618 0.57735026918962518]  FollAlignAxisA=+X  BaseAlignAxisA=+Y  FollAlignAxisB=+Y  BaseAlignAxisB=+Z  BlockFunction=simmechanics.library.frames_transforms.rigid_transform
  Transform1 : sm_lib/Frames and Transforms/Rigid Transform  TranslationMethod=None  TranslationLengthUnit=mm  TranslationStandardAxis=+Z  TranslationStandardOffset=0  TranslationCartesianOffset=[1.3358203432289883e-12 0 -1.0913936421275139e-11]  TranslationROffset=0  TranslationROffsetUnits=m  TranslationZOffset=0  TranslationZOffsetUnits=m  TranslationThetaOffset=0  TranslationThetaOffsetUnits=deg  RotationMethod=None  RotationAngleUnits=rad  RotationStandardAxis=+X  RotationAngle=pi/2  RotationArbitraryAxis=[0 0 0]  FollAlignAxisA=+X  BaseAlignAxisA=+Y  FollAlignAxisB=+Y  BaseAlignAxisB=+Z  BlockFunction=simmechanics.library.frames_transforms.rigid_transform
  F : PMIOPort  Port=1  Side=Right
  B : PMIOPort  Port=2  Side=Left
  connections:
  Transform/LConn1 -- Transform1/LConn1 -- ReferenceFrame/RConn1 -- Solid/RConn1
  Transform/RConn1 -- B/RConn1
  Transform1/RConn1 -- F/RConn1

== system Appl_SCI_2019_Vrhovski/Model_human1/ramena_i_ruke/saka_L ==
  ReferenceFrame : sm_lib/Frames and Transforms/Reference Frame  BlockFunction=simmechanics.library.frames_transforms.reference_frame
  Solid : sm_lib/Body Elements/Solid  InertiaType=Custom  Mass=0  MassUnits=kg  CenterOfMass=[0 0 0]  CenterOfMassUnits=mm  MomentsOfInertia=[2897.1863857204326 1.8962829928219973 2897.1862300567827]  MomentsOfInertiaUnits=kg*mm^2  ProductsOfInertia=[0 0 -0.00027890183916846033]  ProductsOfInertiaUnits=kg*mm^2  DensityBased=on  Density=1000  DensityUnits=kg/(m^3)  GraphicType=FromGeometry  MarkerShape=Sphere  MarkerSize=10  MarkerSizeUnits=m  GraphicVisPropType=SimpleVisualProperties  GraphicDiffuseColor=[0.792156862745098 0.81960784313725488 0.93333333333333335]  GraphicSpecularColor=[0.5 0.5 0.5 1.0]  GraphicAmbientColor=[0.15 0.15 0.15 1.0]  GraphicEmissiveColor=[0.0 0.0 0.0 1.0]  GraphicShininess=75  GraphicOpacity=1  GeometryShape=Sphere  RectangleSize=[1 1]  RectangleSizeUnits=m  BrickDimensions=[1 1 1]  BrickDimensionUnits=m  CylinderRadius=1  CylinderRadiusUnits=m  CylinderLength=1  CylinderLengthUnits=m  SphereRadius=3  SphereRadiusUnits=cm  EllipsoidRadii=[1 1 1]  EllipsoidRadiiUnits=m  ExtrusionCrossSection=[1 1; -1 1; -1 -1; 1 -1]  ExtrusionCrossSectionUnits=m  ExtrusionLength=1  ExtrusionLengthUnits=m  PolygonNumSides=3  PolygonOuterRadius=1  PolygonOuterRadiusUnits=m  ExtGeomFileType=STL  ExtGeomFileName=Pod_Default_sldprt.STL  ExtGeomFileUnits=mm  RevolutionCrossSection=[1 1; 1 -1; 2 -1; 2 1]  RevolutionCrossSectionUnits=m  RevolutionExtent=Full  RevolutionAngle=180  RevolutionAngleUnits=deg  BlockFunction=simmechanics.library.body_elements.solid
  Transform : sm_lib/Frames and Transforms/Rigid Transform  TranslationMethod=None  TranslationLengthUnit=mm  TranslationStandardAxis=+Z  TranslationStandardOffset=0  TranslationCartesianOffset=[-2.2026824808563106e-13 549.99999999999943 3.4106051316484809e-13]  TranslationROffset=0  TranslationROffsetUnits=m  TranslationZOffset=0  TranslationZOffsetUnits=m  TranslationThetaOffset=0  TranslationThetaOffsetUnits=deg  RotationMethod=None  RotationAngleUnits=rad  RotationStandardAxis=+Z  RotationAngle=2.0943951023931962  RotationArbitraryAxis=[0.57735026918962595 -0.57735026918962618 0.57735026918962518]  FollAlignAxisA=+X  BaseAlignAxisA=+Y  FollAlignAxisB=+Y  BaseAlignAxisB=+Z  BlockFunction=simmechanics.library.frames_transforms.rigid_transform
  Transform1 : sm_lib/Frames and Transforms/Rigid Transform  TranslationMethod=None  TranslationLengthUnit=mm  TranslationStandardAxis=+Z  TranslationStandardOffset=0  TranslationCartesianOffset=[1.3358203432289883e-12 0 -1.0913936421275139e-11]  TranslationROffset=0  TranslationROffsetUnits=m  TranslationZOffset=0  TranslationZOffsetUnits=m  TranslationThetaOffset=0  TranslationThetaOffsetUnits=deg  RotationMethod=None  RotationAngleUnits=rad  RotationStandardAxis=+X  RotationAngle=pi/2  RotationArbitraryAxis=[0 0 0]  FollAlignAxisA=+X  BaseAlignAxisA=+Y  FollAlignAxisB=+Y  BaseAlignAxisB=+Z  BlockFunction=simmechanics.library.frames_transforms.rigid_transform
  F : PMIOPort  Port=1  Side=Right
  B : PMIOPort  Port=2  Side=Left
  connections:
  Transform1/RConn1 -- F/RConn1
  Transform/RConn1 -- B/RConn1
  Solid/RConn1 -- ReferenceFrame/RConn1 -- Transform1/LConn1 -- Transform/LConn1

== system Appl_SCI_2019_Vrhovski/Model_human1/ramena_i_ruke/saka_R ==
  ReferenceFrame : sm_lib/Frames and Transforms/Reference Frame  BlockFunction=simmechanics.library.frames_transforms.reference_frame
  Solid : sm_lib/Body Elements/Solid  InertiaType=Custom  Mass=0  MassUnits=kg  CenterOfMass=[0 0 0]  CenterOfMassUnits=mm  MomentsOfInertia=[2897.1863857204326 1.8962829928219973 2897.1862300567827]  MomentsOfInertiaUnits=kg*mm^2  ProductsOfInertia=[0 0 -0.00027890183916846033]  ProductsOfInertiaUnits=kg*mm^2  DensityBased=on  Density=1000  DensityUnits=kg/(m^3)  GraphicType=FromGeometry  MarkerShape=Sphere  MarkerSize=10  MarkerSizeUnits=m  GraphicVisPropType=SimpleVisualProperties  GraphicDiffuseColor=[0.792156862745098 0.81960784313725488 0.93333333333333335]  GraphicSpecularColor=[0.5 0.5 0.5 1.0]  GraphicAmbientColor=[0.15 0.15 0.15 1.0]  GraphicEmissiveColor=[0.0 0.0 0.0 1.0]  GraphicShininess=75  GraphicOpacity=1  GeometryShape=Sphere  RectangleSize=[1 1]  RectangleSizeUnits=m  BrickDimensions=[1 1 1]  BrickDimensionUnits=m  CylinderRadius=1  CylinderRadiusUnits=m  CylinderLength=1  CylinderLengthUnits=m  SphereRadius=3  SphereRadiusUnits=cm  EllipsoidRadii=[1 1 1]  EllipsoidRadiiUnits=m  ExtrusionCrossSection=[1 1; -1 1; -1 -1; 1 -1]  ExtrusionCrossSectionUnits=m  ExtrusionLength=1  ExtrusionLengthUnits=m  PolygonNumSides=3  PolygonOuterRadius=1  PolygonOuterRadiusUnits=m  ExtGeomFileType=STL  ExtGeomFileName=Pod_Default_sldprt.STL  ExtGeomFileUnits=mm  RevolutionCrossSection=[1 1; 1 -1; 2 -1; 2 1]  RevolutionCrossSectionUnits=m  RevolutionExtent=Full  RevolutionAngle=180  RevolutionAngleUnits=deg  BlockFunction=simmechanics.library.body_elements.solid
  Transform : sm_lib/Frames and Transforms/Rigid Transform  TranslationMethod=None  TranslationLengthUnit=mm  TranslationStandardAxis=+Z  TranslationStandardOffset=0  TranslationCartesianOffset=[-2.2026824808563106e-13 549.99999999999943 3.4106051316484809e-13]  TranslationROffset=0  TranslationROffsetUnits=m  TranslationZOffset=0  TranslationZOffsetUnits=m  TranslationThetaOffset=0  TranslationThetaOffsetUnits=deg  RotationMethod=None  RotationAngleUnits=rad  RotationStandardAxis=+Z  RotationAngle=2.0943951023931962  RotationArbitraryAxis=[0.57735026918962595 -0.57735026918962618 0.57735026918962518]  FollAlignAxisA=+X  BaseAlignAxisA=+Y  FollAlignAxisB=+Y  BaseAlignAxisB=+Z  BlockFunction=simmechanics.library.frames_transforms.rigid_transform
  Transform1 : sm_lib/Frames and Transforms/Rigid Transform  TranslationMethod=None  TranslationLengthUnit=mm  TranslationStandardAxis=+Z  TranslationStandardOffset=0  TranslationCartesianOffset=[1.3358203432289883e-12 0 -1.0913936421275139e-11]  TranslationROffset=0  TranslationROffsetUnits=m  TranslationZOffset=0  TranslationZOffsetUnits=m  TranslationThetaOffset=0  TranslationThetaOffsetUnits=deg  RotationMethod=None  RotationAngleUnits=rad  RotationStandardAxis=+X  RotationAngle=pi/2  RotationArbitraryAxis=[0 0 0]  FollAlignAxisA=+X  BaseAlignAxisA=+Y  FollAlignAxisB=+Y  BaseAlignAxisB=+Z  BlockFunction=simmechanics.library.frames_transforms.rigid_transform
  F : PMIOPort  Port=1  Side=Right
  B : PMIOPort  Port=2  Side=Left
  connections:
  Transform/LConn1 -- Transform1/LConn1 -- ReferenceFrame/RConn1 -- Solid/RConn1
  Transform/RConn1 -- B/RConn1
  Transform1/RConn1 -- F/RConn1
